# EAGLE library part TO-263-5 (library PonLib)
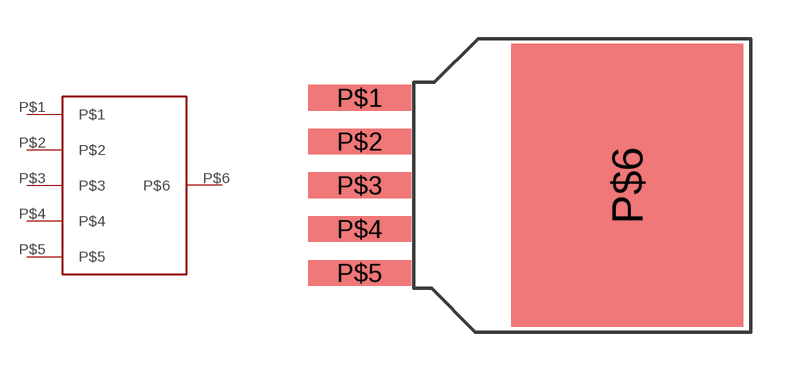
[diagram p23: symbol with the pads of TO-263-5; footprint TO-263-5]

Designator prefix -

## TO-263-5  [TO-263-5]
P$1  P$1
P$2  P$2
P$3  P$3
P$4  P$4
P$5  P$5
P$6  P$6

## Footprint TO-263-5 (pad centres in mm)
smd 4 x 1: P$1 -2,3.4; P$2 -2,1.7; P$3 -2,0; P$4 -2,-1.7; P$5 -2,-3.4
smd 9 x 11: P$6 8.4,0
